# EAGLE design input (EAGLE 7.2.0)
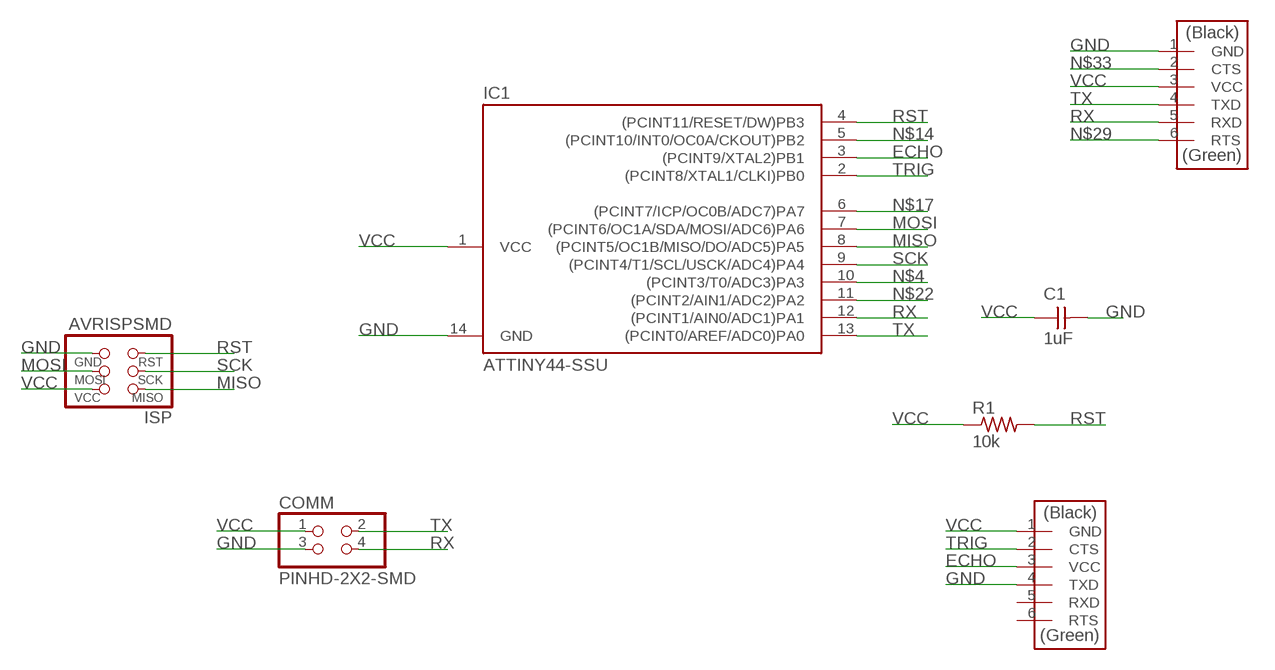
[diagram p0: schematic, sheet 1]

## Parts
C1  1uF  CAP-UNPOLARIZEDFAB  [C1206FAB]
COMM  PINHD-2X2-SMD  [2X02SMD]
FTDI  FTDI-SMD-HEADER  [1X06SMD]
IC1  ATTINY44-SSU  [SOIC14]
ISP  AVRISPSMD  [2X03SMD]
R1  10k  RES-US1206FAB  [R1206FAB]
SENSOR  FTDI-SMD-HEADER  [1X06SMD]

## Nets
ECHO: IC1.3((PCINT9/XTAL2)PB1) SENSOR.3(VCC)
GND: C1.2 COMM.3 FTDI.1(GND) IC1.14(GND) ISP.6(GND) SENSOR.4(TXD)
MISO: IC1.8((PCINT5/OC1B/MISO/DO/ADC5)PA5) ISP.1(MISO)
MOSI: IC1.7((PCINT6/OC1A/SDA/MOSI/ADC6)PA6) ISP.4(MOSI)
N$4: IC1.10((PCINT3/T0/ADC3)PA3)
N$14: IC1.5((PCINT10/INT0/OC0A/CKOUT)PB2)
N$17: IC1.6((PCINT7/ICP/OC0B/ADC7)PA7)
N$22: IC1.11((PCINT2/AIN1/ADC2)PA2)
N$29: FTDI.6(RTS)
N$33: FTDI.2(CTS)
RST: IC1.4((PCINT11/RESET/DW)PB3) ISP.5(RST) R1.2
RX: COMM.4 FTDI.5(RXD) IC1.12((PCINT1/AIN0/ADC1)PA1)
SCK: IC1.9((PCINT4/T1/SCL/USCK/ADC4)PA4) ISP.3(SCK)
TRIG: IC1.2((PCINT8/XTAL1/CLKI)PB0) SENSOR.2(CTS)
TX: COMM.2 FTDI.4(TXD) IC1.13((PCINT0/AREF/ADC0)PA0)
VCC: C1.1 COMM.1 FTDI.3(VCC) IC1.1(VCC) ISP.2(VCC) R1.1 SENSOR.1(GND)
Unconnected: SENSOR.5(RXD) SENSOR.6(RTS)

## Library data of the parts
C1 = fab:CAP-UNPOLARIZED
COMM = fab:PINHD-2X2-SMD
FTDI SENSOR = fab:FTDI-SMD-HEADER
IC1 = fab:ATTINY44
ISP = fab:AVRISP
R1 = fab:RES-US: Resistor (US Symbol)

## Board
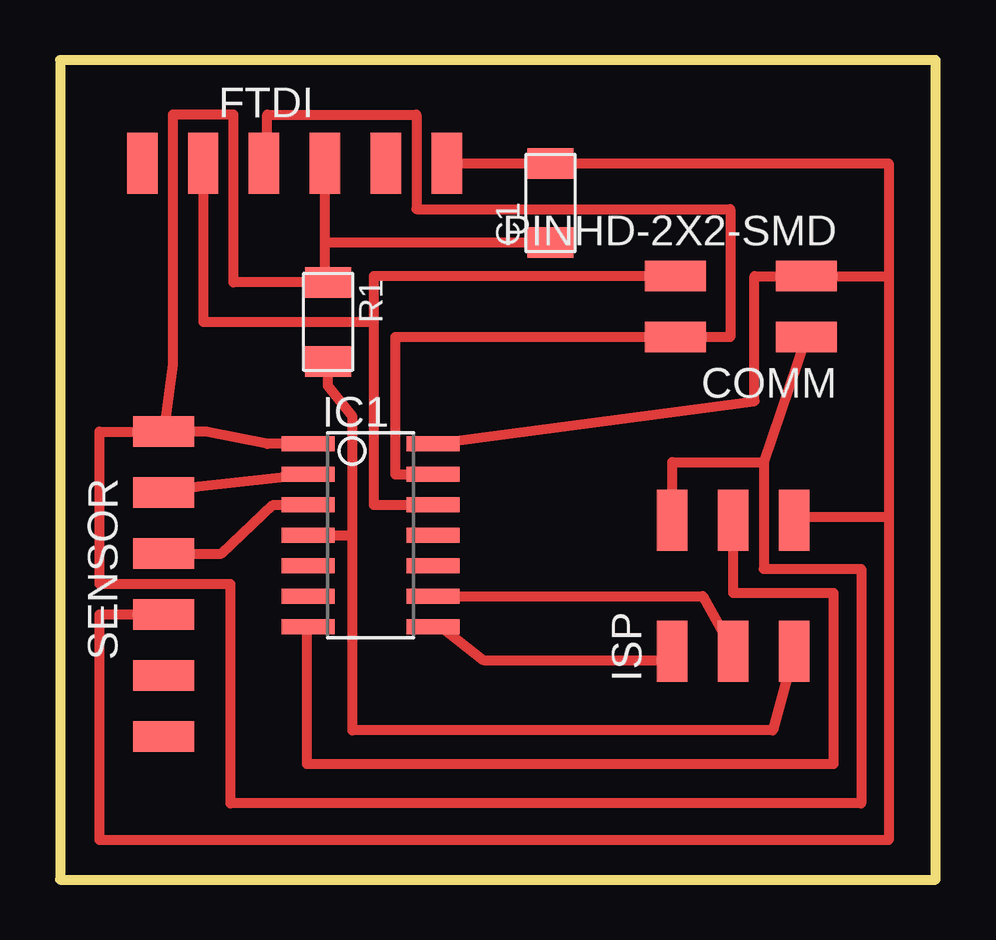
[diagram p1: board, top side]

Size 36.5 x 34.15 mm. Coordinates in mm from the lower left corner, seen from the top.
Outline: 0,0 36.5,0 36.5,34.15 0,34.15 0,0
Copper layers (1*16): Top 0.035mm / dielectric 1.5mm / Bottom 0.035mm
Design rules "default": minimum track width 10mil, minimum drill 24mil, track to track 8mil, track to pad 8mil, pad to pad 8mil, via to via 8mil, smd to smd 8mil, copper to edge 40mil, drill to drill 8mil, minimum pad ring 10mil, minimum via ring 8mil, stop-mask expansion 4mil, vias tented up to drill 0mil, thermal gap 10mil

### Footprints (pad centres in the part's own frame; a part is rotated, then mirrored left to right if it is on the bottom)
C1206FAB = smd 1.27 x 1.905: 1 -1.651,0; 2 1.651,0
2X02SMD = smd 2.54 x 1.27: 1 -2.54,1.27; 2 2.92,1.27; 3 -2.54,-1.27; 4 2.92,-1.27
1X06SMD = smd 2.54 x 1.27: 1 0,6.35; 2 0,3.81; 3 0,1.27; 4 0,-1.27; 5 0,-3.81; 6 0,-6.35
SOIC14 = smd 0.61 x 2.21: 1 -3.81,-2.603; 2 -2.54,-2.603; 3 -1.27,-2.603; 4 0,-2.603; 5 1.27,-2.603; 6 2.54,-2.603; 7 3.81,-2.603; 8 3.81,2.603; 9 2.54,2.603; 10 1.27,2.603; 11 0,2.603; 12 -1.27,2.603; 13 -2.54,2.603; 14 -3.81,2.603
2X03SMD = smd 2.54 x 1.27: 1 -2.54,2.54; 2 2.92,2.54; 3 -2.54,0; 4 2.92,0; 5 -2.54,-2.54; 6 2.92,-2.54
R1206FAB = smd 1.27 x 1.905: 1 -1.651,0; 2 1.651,0

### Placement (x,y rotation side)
C1  20.45,28.19 90 top
COMM  28.57,23.88 180 top
FTDI  9.78,29.84 270 top
IC1  12.95,14.35 270 top
ISP  28.07,12.06 90 top
R1  11.18,23.24 270 top
SENSOR  4.32,12.32 0 top

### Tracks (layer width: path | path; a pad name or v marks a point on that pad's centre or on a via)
ECHO
  Top 0.406: SENSOR.3 6.73,13.59 8.89,15.62 IC1.3
GND
  Top 0.406: FTDI.1 C1.2 34.54,29.84 34.54,25.15 | 34.54,25.15 34.54,15.11 | 34.54,15.11 34.54,1.65 1.65,1.65 1.65,11.05 SENSOR.4 | 34.54,25.15 COMM.3 28.96,25.15 28.96,19.94 IC1.14 | ISP.6 30.73,14.98 30.73,15.11 34.54,15.11
MISO
  Top 0.406: IC1.8 15.88,10.54 17.65,9.14 25.53,9.14 ISP.1
MOSI
  Top 0.406: IC1.7 10.29,10.54 10.29,4.83 32.26,4.83 32.26,11.94 28.07,11.94 ISP.4
RST
  Top 0.406: IC1.4 12.19,14.35 | 12.19,14.35 12.19,19.3 11.18,20.57 R1.2 | ISP.5 29.72,6.22 12.19,6.22 12.19,14.35
RX
  Top 0.406: FTDI.5 5.97,23.24 13.08,23.24 | 13.08,23.24 13.08,15.62 IC1.12 | COMM.4 13.08,25.15 13.08,23.24
SCK
  Top 0.406: IC1.9 26.8,11.81 ISP.3
TRIG
  Top 0.406: SENSOR.2 5.78,16.38 IC1.2
TX
  Top 0.406: FTDI.4 8.64,29.84 8.64,31.88 14.86,31.88 14.86,27.94 27.94,27.94 27.94,22.61 COMM.2 13.97,22.61 13.97,16.89 IC1.13
VCC
  Top 0.406: 11.05,26.54 11.05,24.89 R1.1 7.24,24.89 7.24,31.88 4.7,31.88 4.7,21.46 SENSOR.1 | 11.05,26.54 FTDI.3 | C1.1 11.05,26.54 | IC1.1 8.64,18.16 6.1,18.67 SENSOR.1 | ISP.2 25.53,17.4 29.34,17.4 | 29.34,17.4 29.34,12.95 33.4,12.95 33.4,3.17 7.11,3.17 7.11,12.32 1.65,12.32 1.65,18.67 SENSOR.1 | COMM.1 29.34,17.4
